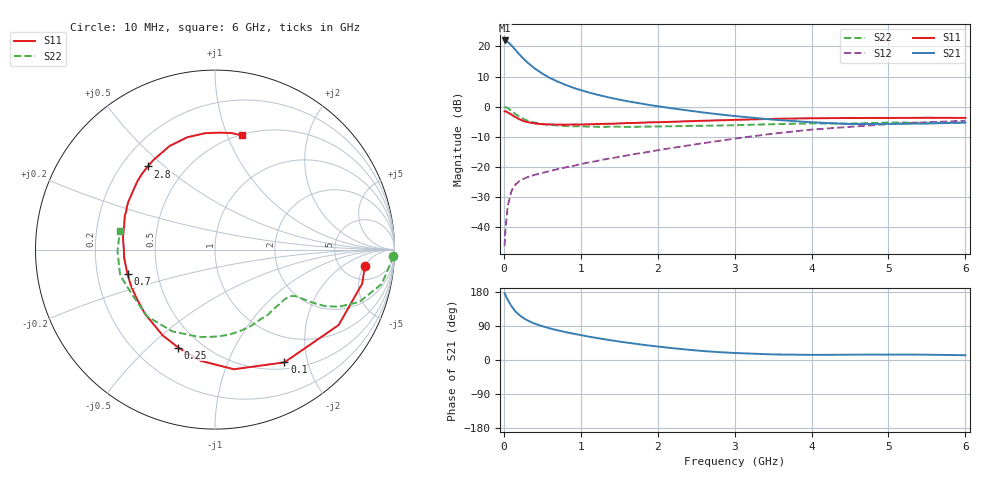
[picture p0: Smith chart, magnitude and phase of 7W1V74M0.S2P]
! Infineon Technologies  Discrete & RF Semiconductors
! BFS17W
! Si NPN RF Bipolar Junction Transistor in SOT323
! VCE = 1.75 V  IC = 4 mA
! Common Emitter S-Parameters:  August  1999
# GHz  S  MA  R  50
!  f  S11  S21  S12  S22
! GHz  MAG  ANG  MAG  ANG  MAG  ANG  MAG  ANG
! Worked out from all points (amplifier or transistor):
!   36 points, 10 MHz to 6 GHz, reference 50 ohm
!   highest |S21| = 22.0 dB at 10 MHz (marker M1)
!   |S21| within 3 dB of that: start of sweep to 146.6 MHz
!   unconditionally stable (mu >= 1): 584.6 MHz to end of sweep
!   at 250 MHz: K = 0.53, MSG = 20.0 dB, |S12| = -24.0 dB
!   at 1.4 GHz: K = 1.31, MAG = 6.6 dB, |S12| = -17.1 dB
!   at 6 GHz: K = 1.10, MAG = -2.3 dB, |S12| = -4.6 dB
!   S11 on the Smith chart (normalised r, x): 10 MHz: 8.16, -5.19; 100 MHz: 0.59, -1.63; 250 MHz: 0.38, -0.62; 700 MHz: 0.33, -0.12; 2.8 GHz: 0.31, +0.44; 6 GHz: 0.51, +1.13
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0.01  0.84 -6.4  12.54 176.3  0.0049 85.2  0.9939 -1.9
0.02  0.8418 -13.0  12.4 171.5  0.009 87.4  0.9791 -4.8
0.05  0.807 -31.4  11.91 159.0  0.0227 76.3  0.9489 -11.6
0.1  0.7377 -58.4  10.35 141.9  0.0404 62.1  0.8547 -20.0
0.15  0.6749 -81.0  8.777 128.3  0.0513 53.5  0.7598 -24.8
0.2  0.6247 -97.3  7.422 118.7  0.0587 48.8  0.688 -27.2
0.25  0.5828 -110.6  6.342 111.2  0.0634 45.7  0.6316 -28.3
0.3  0.5599 -121.4  5.5 105.3  0.0676 44.4  0.5945 -28.9
0.4  0.5293 -137.6  4.325 96.0  0.0743 43.6  0.5446 -29.5
0.5  0.5137 -148.9  3.543 89.2  0.0801 44.7  0.5178 -30.0
0.6  0.509 -157.5  2.994 83.3  0.086 46.3  0.5005 -31.1
0.7  0.5063 -164.3  2.609 78.3  0.0927 48.1  0.4893 -32.6
0.9  0.5087 -175.3  2.07 69.6  0.1046 50.7  0.4747 -36.4
1.1  0.5124 175.6  1.73 61.8  0.1192 53.3  0.4691 -41.3
1.3  0.5204 168.2  1.491 55.0  0.1338 55.1  0.4644 -46.8
1.6  0.5371 159.2  1.238 45.8  0.1561 57.4  0.4636 -55.3
2.2  0.5635 143.5  0.937 31.0  0.2092 59.8  0.4759 -74.3
2.8  0.5958 129.0  0.748 20.7  0.2719 58.9  0.4882 -94.3
3.5  0.6303 113.6  0.611 14.7  0.3587 54.3  0.514 -117.6
4.5  0.651 94.9  0.517 14.0  0.4646 42.5  0.5253 -151.3
5.5  0.656 81.8  0.527 14.0  0.5521 30.7  0.5432 -179.0
6  0.6537 76.7  0.548 12.6  0.5863 25.1  0.5405 168.8
